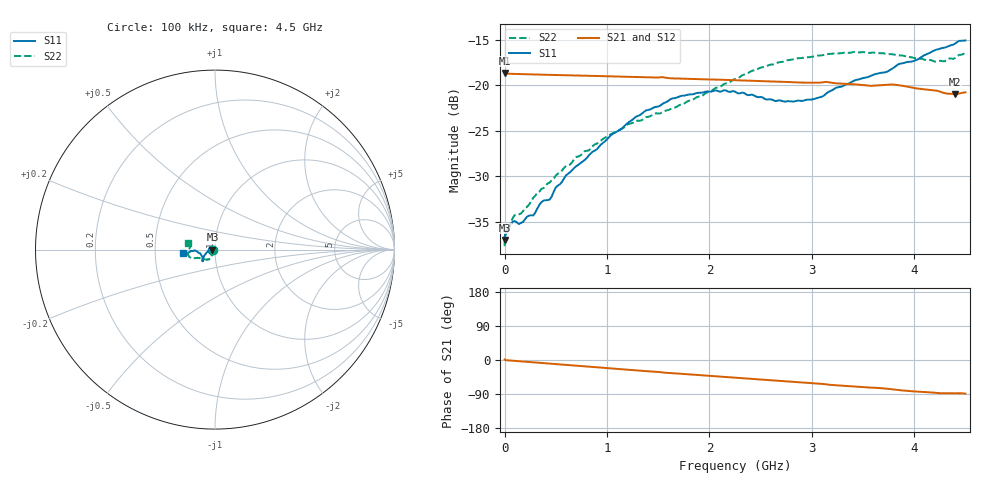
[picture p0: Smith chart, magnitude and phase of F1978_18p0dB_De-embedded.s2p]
! Integrated Device Technology
! Corporate Headquarters
! 6024 Silver Creek Valley Road
! San Jose, CA 95138  USA
! Phone:  1-408-284-8200
! Toll Free:  1-800-223-1366
! Webpage:  http://www.idt.com/
! Timing and RF Division
! 515 Groton Road, Suite 102
! Westford, MA 01886-6024
! Device:  F1978
! Description: 6-bit, 75 ohm, 0.5 dB Digital Step Attenuator
! Frequency:  5.0 MHz -  3.00 GHz
! Package:  4x4 mm QFN Plastic Package: 20 pin
! Ports:  2 RF, 11 DC
!  Pin  1  = D5 (16 dB)
!  Pin  2  = RF1  =  Port 1
!  Pin  3  = Serial Data In (DATA)
!  Pin  4  = Serial Clock (CLK)
!  Pin  5  = Serial Latch Enable (LE)
!  Pin  6  = VDD
!  Pin  7  = NC
!  Pin  8  = NC
!  Pin  9  = NC
!  Pin 10  = GND
!  Pin 11  = GND
!  Pin 12  = NC
!  Pin 13  = VMODE
!  Pin 14  = RF2  =  Port 2
!  Pin 15  = D4 (8 dB)
!  Pin 16  = D3 (4 dB)
!  Pin 17  = D2 (2 dB)
!  Pin 18  = NC
!  Pin 19  = D1 (1 dB)
!  Pin 20  = D0 (0.5 dB)
! State:  36
! Atten State:  18.0 dB
! Voltage:  +3.30 Volts
! Current:  0.593 mA
! Data:  The device was measured on a F1975 evaluation board which has
!  individual transmission lines to the RF pins.  Data was collected
!  using a calibrated network analyzer.  The evaluation board was
!  de-embedded using Automatic Fixture Removal (AFR).
!  The reference plane is the edge of the package pin.
! Misc:
!  Action Tracker AT0416
! Date Measured:  2018-02-08
! Date:  2018-03-26  MJV
! Note:
!  Integrated Device Technology supplies this data as a sample of measured
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# GHz S dB R 75
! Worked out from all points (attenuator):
!   291 points, 100 kHz to 4.5 GHz, reference 75 ohm
!   highest |S21| = -18.61 dB at 100 kHz (marker M1); lowest = -21.0 dB at 4.4 GHz (marker M2)
!   lowest |S11| = -37.0 dB at 100 kHz (marker M3), VSWR 1.03, Z = 72.9 + j0.00149 ohm
!   |S11| at or under -10 dB: start of sweep to end of sweep
!   |S22| runs from -37.7 to -16.3 dB; largest |S21 - S12| = 0.00021
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0.0001  -36.99 180.0  -18.61 1.2  -18.61 1.2  -37.69 -178.2
0.0009  -36.69 -177.9  -18.64 1.1  -18.64 1.0  -36.98 -177.3
0.01  -36.32 -177.9  -18.68 -0.4  -18.68 -0.4  -36.37 -174.0
0.1  -34.92 -174.2  -18.73 -2.5  -18.73 -2.5  -34.26 -155.6
0.16  -35.13 -175.9  -18.75 -3.8  -18.75 -3.8  -34.10 -145.9
0.28  -34.30 -177.8  -18.79 -6.4  -18.78 -6.4  -32.36 -135.5
0.36  -32.85 -177.8  -18.81 -8.1  -18.81 -8.1  -31.38 -127.8
0.44  -32.55 -176.9  -18.83 -9.7  -18.82 -9.8  -30.69 -122.6
0.5  -31.22 -177.2  -18.84 -11.0  -18.84 -11.0  -29.91 -122.5
0.6  -29.89 -173.4  -18.87 -13.1  -18.87 -13.1  -28.85 -119.1
0.76  -28.39 -166.5  -18.91 -16.5  -18.91 -16.5  -27.47 -117.8
1.28  -23.47 -151.0  -19.07 -27.3  -19.07 -27.3  -23.92 -120.9
1.52  -22.21 -144.4  -19.09 -32.0  -19.09 -32.0  -23.07 -128.1
1.88  -20.82 -138.2  -19.30 -39.4  -19.29 -39.4  -21.27 -143.0
2.26  -20.74 -137.4  -19.41 -46.9  -19.41 -46.9  -19.26 -154.6
2.64  -21.71 -148.0  -19.56 -54.4  -19.56 -54.4  -17.61 -158.8
3.02  -21.49 -164.5  -19.69 -61.6  -19.68 -61.6  -16.79 -162.4
3.42  -19.44 -175.8  -19.88 -70.3  -19.88 -70.3  -16.31 -169.1
3.76  -18.33 -176.2  -19.89 -76.5  -19.89 -76.5  -16.55 -176.3
4.2  -16.13 -173.3  -20.54 -86.4  -20.54 -86.4  -17.37 171.3
4.4  -15.38 -171.2  -20.95 -87.9  -20.95 -87.8  -16.97 168.0
4.5  -15.04 -173.0  -20.75 -88.7  -20.74 -88.7  -16.35 166.7
